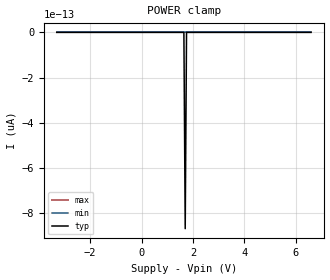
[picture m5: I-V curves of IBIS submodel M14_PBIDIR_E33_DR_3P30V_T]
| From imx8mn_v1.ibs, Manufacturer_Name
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| Submodel
[Submodel]  M14_PBIDIR_E33_DR_3P30V_T
Submodel_type Dynamic_clamp
[POWER Clamp]
| Voltage   I(typ)   I(min)   I(max)
-3.3V     0A         0A         0A
1.65V     0A         0A         0A
1.702V    0A         0A         0A
1.753V    0A         0A         0A
6.6V      0A         0A         0A
